[IBIS Ver]   4.2
[File Name]  stm32f2_wlcsp64.ibs
[File Rev]   1.0
[Date]   31-Aug-2011
[Source]   STMicroelectronics NV
[Notes]   The I/O models have been made by simulation and qualified
   with recomandation of QualityIBIS flow.
   Some Models, library and pin names may be modified.
   Details of modified names can be found below.
ORIGINAL NAME   ::  MODIFIED NAME   :: COMMENTS(if any)
IO8USB_LSFS_OTG_FT  ::  IO8USB_LSFS_OTG_FT_USB   :: Model in USB mode.
IO8USB_LSFS_OTG_FT  ::  IO8USB_LSFS_OTG_FT_NON_USB_DNV33  :: Model in other than USB mode & pad pin = DNV33
IO8USB_LSFS_OTG_FT  ::  IO8USB_LSFS_OTG_FT_NON_USB_DPV33  :: Model in other than USB mode & pad pin = DPV33
[Disclaimer] These IBIS models are the proprietary information of
   STMicroelectronics and are disclosed to users solely for
   modeling and simulation purposes. No further license is
   implied. All warranties express, implied, or statutory,
   including any implied warranty of fitness for a particular
   purpose or implied warranty against infringement, are
   hereby disclaimed. STMicroelectronics reserves the right
   to change the IBIS models at any time and without notice.
[Copyright]  (c) STMicroelectronics
   All rights reserved. Reproduction in whole or part is prohibited
   without the written consent of the copyright holder.
[Component]  STM32F2_WLCSP
[Manufacturer] STMicroelectronics NV
[Package]
| variable   typ   min   max
R_pkg   0.000mOhm   0.000mOhm   0.000mOhm
L_pkg   0.000nH   0.000nH   0.000nH
C_pkg   0.000pF   0.000pF   0.000pF
[Pin]   signal_name   model_name
|- PE2 IO8PROG2M25M50M100M_ARSUDQ_FT
|- PE3 IO8PROG2M25M50M100M_ARSUDQ_FT
|- PE4 IO8PROG2M25M50M100M_ARSUDQ_FT
|- PE5 IO8PROG2M25M50M100M_ARSUDQ_FT
|- PE6 IO8PROG2M25M50M100M_ARSUDQ_FT
|A9 VBAT VDD33IOSWCO_MOSSWI_FT
B8 PC13 IO8PROG2M25M50M100M_ARWSUDQ_FT_V33
B9 PC14 IO8PROG2M25M50M100M_ARWSUDQ_FT
C9 PC15 IO8PROG2M25M50M100M_ARSUDQ_FT
|- VSS_5 VSSIOCO
|- VDD_5 VDD33IOCO
E9 PH0 IO8PROG2M25M50M100M_ARSUDQ_FT
F9 PH1 IO8PROG2M25M50M100M_ARSUDQ_FT
|E8 NRST RESET
G9 PC0 IO8PROG2M25M50M100M_AR3WSUDQ_FT
F8 PC1 IO8PROG2M25M50M100M_AR3WSUDQ_FT
D7 PC2 IO8PROG2M25M50M100M_AR3WSUDQ_FT
G8 PC3 IO8PROG2M25M50M100M_AR3WSUDQ_FT
|- VDD_12 VDD33IOCO_VSSIOCO_MOSSWI_FT
|- VSSA VSSCO
|F7 VREF+ VDD33CO
|- VDDA VDD33CO
E7 PA0 IO8PROG2M25M50M100M_AR3WSUDQ_FT_V33
H8 PA1 IO8PROG2M25M50M100M_AR3WSUDQ_FT
J9 PA2 IO8PROG2M25M50M100M_AR3WSUDQ_FT
G7 PA3 IO8PROG2M25M50M100M_AR3WSUDQ_FT
|F1 VSS_4 VSSIOCO
|H7 REGOFF VSSIOCO
|E1 VDD_4 VDD33IOCO
J8 PA4 IO8PROG2M25M50M100M_AR3WSUDQ_FT
H6 PA5 IO8PROG2M25M50M100M_AR3WSUDQ_FT
H5 PA6 IO8PROG2M25M50M100M_AR3WSUDQ_FT
J7 PA7 IO8PROG2M25M50M100M_AR3WSUDQ_FT
H4 PC4 IO8PROG2M25M50M100M_AR3WSUDQ_FT
G3 PC5 IO8PROG2M25M50M100M_AR3WSUDQ_FT
J6 PB0 IO8PROG2M25M50M100M_AR3WSUDQ_FT
J5 PB1 IO8PROG2M25M50M100M_AR3WSUDQ_FT
J4 PB2 IO8PROG2M25M50M100M_AR3WSUDQ_FT
|- PE7 IO8PROG2M25M50M100M_ARSUDQ_FT
|- PE8 IO8PROG2M25M50M100M_ARSUDQ_FT
|- PE9 IO8PROG2M25M50M100M_ARSUDQ_FT
|- PE10 IO8PROG2M25M50M100M_ARSUDQ_FT
|- PE11 IO8PROG2M25M50M100M_ARSUDQ_FT
|- PE12 IO8PROG2M25M50M100M_ARSUDQ_FT
|- PE13 IO8PROG2M25M50M100M_ARSUDQ_FT
|- PE14 IO8PROG2M25M50M100M_ARSUDQ_FT
|- PE15 IO8PROG2M25M50M100M_ARSUDQ_FT
H3 PB10 IO8PROG2M25M50M100M_ARSUDQ_I2CIN_FT
J2 PB11 IO8PROG2M25M50M100M_ARSUDQ_I2CIN_FT
|J3 VCAP1_0
|- VDD_1
J1 PB12 IO8USB_ID_OTG_FT
H2 PB13 IO8USB_VBUS_OTG_FT
|H1 PA11 IO8USB_LSFS_OTG_FT_USB
H1 PA11 IO8USB_LSFS_OTG_FT_NON_USB_DNV33
|G1 PA12 IO8USB_LSFS_OTG_FT_USB
G1 PA12 IO8USB_LSFS_OTG_FT_NON_USB_DPV33
|- PD8 IO8PROG2M25M50M100M_ARSUDQ_FT
|- PD9 IO8PROG2M25M50M100M_ARSUDQ_FT
|- PD10 IO8PROG2M25M50M100M_ARSUDQ_FT
|- PD11 IO8PROG2M25M50M100M_ARSUDQ_FT
|- PD12 IO8PROG2M25M50M100M_ARSUDQ_FT
|- PD13 IO8PROG2M25M50M100M_ARSUDQ_FT
|- PD14 IO8PROG2M25M50M100M_ARSUDQ_FT
|- PD15 IO8PROG2M25M50M100M_ARSUDQ_FT
G2 PC6 IO8PROG2M25M50M100M_ARSUDQ_FT
F2 PC7 IO8PROG2M25M50M100M_ARSUDQ_FT
F3 PC8 IO8PROG2M25M50M100M_ARSUDQ_FT
D1 PC9 IO8PROG2M25M50M100M_ARSUDQ_I2CIN_FT
E2 PA8 IO8PROG2M25M50M100M_ARSUDQ_I2CIN_FT
E3 PA9 IO8USB_VBUS_OTG_FT
D3 PA10 IO8USB_ID_OTG_FT
D2 PA11 IO8USB_LSFS_OTG_FT_USB
|D2 PA11 IO8USB_LSFS_OTG_FT_NON_USB_DNV33
C1 PA12 IO8USB_LSFS_OTG_FT_USB
|C1 PA12 IO8USB_LSFS_OTG_FT_NON_USB_DPV33
B2 PA13 IO8PROG2M25M50M100M_ARSUDQ_FT
|C2 VCAP2
|B1 VSS_2
|A8 VDD_2
A1 PA14 IO8PROG2M25M50M100M_ARSUDQ_FT
A2 PA15 IO8PROG2M25M50M100M_AR3WSUDQ_FT
B3 PC10 IO8PROG2M25M50M100M_ARSUDQ_FT
C3 PC11 IO8PROG2M25M50M100M_ARSUDQ_FT
A3 PC12 IO8PROG2M25M50M100M_ARSUDQ_FT
|- PD0 IO8PROG2M25M50M100M_ARSUDQ_FT
|- PD1 IO8PROG2M25M50M100M_ARSUDQ_FT
C7 PD2 IO8PROG2M25M50M100M_ARSUDQ_FT
|- PD3 IO8PROG2M25M50M100M_ARSUDQ_FT
|- PD4 IO8PROG2M25M50M100M_ARSUDQ_FT
|- PD5 IO8PROG2M25M50M100M_ARSUDQ_FT
|- PD6 IO8PROG2M25M50M100M_ARSUDQ_FT
|- PD7 IO8PROG2M25M50M100M_ARSUDQ_FT
A4 PB3 IO8PROG2M25M50M100M_ARSUDQ_FT
B4 PB4 IO8PROG2M25M50M100M_ARSUDQ_FT
A5 PB5 IO8PROG2M25M50M100M_AR3WSUDQ_FT
B5 PB6 IO8PROG2M25M50M100M_ARSUDQ_I2CIN_FT
A6 PB7 IO8PROG2M25M50M100M_ARSUDQ_I2CIN_FT
B6 BOOT0 VPP_TEST_HV
B7 PB8 IO8PROG2M25M50M100M_ARSUDQ_I2CIN_FT
A7 PB9 IO8PROG2M25M50M100M_ARSUDQ_I2CIN_FT
|- PE0 IO8PROG2M25M50M100M_ARSUDQ_FT
|- PE1 IO8PROG2M25M50M100M_ARSUDQ_FT
|- NC
|D8 VSS_3
|D9 VDD_3  VDD33CO
[Diff Pin]  inv_pin   vdiff tdelay_typ tdelay_min tdelay_max
H1 G1 200mV 0  0 0
D2 C1 200mV 0  0 0
[Model Selector] IO8PROG2M25M50M100M_AR3WSUDQ_FT_V33
IO8PROG2M25M50M100M_AR3WSUDQ_DRV_V33_00   DRIVER MODEL  : SPEEDAV33=0 SPEEDBV33=0
IO8PROG2M25M50M100M_AR3WSUDQ_DRV_V33_01   DRIVER MODEL  : SPEEDAV33=0 SPEEDBV33=1
IO8PROG2M25M50M100M_AR3WSUDQ_DRV_V33_10   DRIVER MODEL  : SPEEDAV33=1 SPEEDBV33=0
IO8PROG2M25M50M100M_AR3WSUDQ_DRV_V33_11   DRIVER MODEL  : SPEEDAV33=1 SPEEDBV33=1
IO8PROG2M25M50M100M_AR3WSUDQ_RCV_V33_0   CMOS RECIEVER : ENHYSV33=0  OUTPUT=ZIV33
IO8PROG2M25M50M100M_AR3WSUDQ_RCV_V33_0_T  TTL  RECIEVER : ENHYSV33=0  OUTPUT=ZIV33
IO8PROG2M25M50M100M_AR3WSUDQ_RCV_V33_1   CMOS RECIEVER : ENHYSV33=1  OUTPUT=ZIV33
IO8PROG2M25M50M100M_AR3WSUDQ_RCV_V33_1_T  TTL  RECIEVER : ENHYSV33=1  OUTPUT=ZIV33
[Model Selector] IO8PROG2M25M50M100M_AR3WSUDQ_FT
IO8PROG2M25M50M100M_AR3WSUDQ_FT_DRV_00   DRIVER MODEL  : SPEEDAV12=0 SPEEDBV12=0
IO8PROG2M25M50M100M_AR3WSUDQ_FT_DRV_01   DRIVER MODEL  : SPEEDAV12=0 SPEEDBV12=1
IO8PROG2M25M50M100M_AR3WSUDQ_FT_DRV_10   DRIVER MODEL  : SPEEDAV12=1 SPEEDBV12=0
IO8PROG2M25M50M100M_AR3WSUDQ_FT_DRV_11   DRIVER MODEL  : SPEEDAV12=1 SPEEDBV12=1
IO8PROG2M25M50M100M_AR3WSUDQ_FT_RCV_00   CMOS RECIEVER : ENHYSV12=0  OUTPUT=ZIV12
IO8PROG2M25M50M100M_AR3WSUDQ_FT_RCV_00_T  TTL  RECIEVER : ENHYSV12=0  OUTPUT=ZIV12
IO8PROG2M25M50M100M_AR3WSUDQ_FT_RCV_01   CMOS RECIEVER : ENHYSV12=0  OUTPUT=ZIV33
IO8PROG2M25M50M100M_AR3WSUDQ_FT_RCV_01_T  TTL  RECIEVER : ENHYSV12=0  OUTPUT=ZIV33
IO8PROG2M25M50M100M_AR3WSUDQ_FT_RCV_10   CMOS RECIEVER : ENHYSV12=1  OUTPUT=ZIV12
IO8PROG2M25M50M100M_AR3WSUDQ_FT_RCV_10_T  TTL  RECIEVER : ENHYSV12=1  OUTPUT=ZIV12
IO8PROG2M25M50M100M_AR3WSUDQ_FT_RCV_11   CMOS RECIEVER : ENHYSV12=1  OUTPUT=ZIV33
IO8PROG2M25M50M100M_AR3WSUDQ_FT_RCV_11_T  TTL  RECIEVER : ENHYSV12=1  OUTPUT=ZIV33
[Model Selector] IO8PROG2M25M50M100M_ARSUDQ_FT
IO8PROG2M25M50M100M_ARSUDQ_FT_DRV_00   DRIVER MODEL  : SPEEDAV12=0 SPEEDBV12=0
IO8PROG2M25M50M100M_ARSUDQ_FT_DRV_01   DRIVER MODEL  : SPEEDAV12=0 SPEEDBV12=1
IO8PROG2M25M50M100M_ARSUDQ_FT_DRV_10   DRIVER MODEL  : SPEEDAV12=1 SPEEDBV12=0
IO8PROG2M25M50M100M_ARSUDQ_FT_DRV_11   DRIVER MODEL  : SPEEDAV12=1 SPEEDBV12=1
IO8PROG2M25M50M100M_ARSUDQ_FT_RCV_00   CMOS RECIEVER : ENHYSV12=0  OUTPUT=ZIV12
IO8PROG2M25M50M100M_ARSUDQ_FT_RCV_00_T   TTL  RECIEVER : ENHYSV12=0  OUTPUT=ZIV12
IO8PROG2M25M50M100M_ARSUDQ_FT_RCV_01   CMOS RECIEVER : ENHYSV12=0  OUTPUT=ZIV33
IO8PROG2M25M50M100M_ARSUDQ_FT_RCV_01_T   TTL  RECIEVER : ENHYSV12=0  OUTPUT=ZIV33
IO8PROG2M25M50M100M_ARSUDQ_FT_RCV_10   CMOS RECIEVER : ENHYSV12=1  OUTPUT=ZIV12
IO8PROG2M25M50M100M_ARSUDQ_FT_RCV_10_T   TTL  RECIEVER : ENHYSV12=1  OUTPUT=ZIV12
IO8PROG2M25M50M100M_ARSUDQ_FT_RCV_11   CMOS RECIEVER : ENHYSV12=1  OUTPUT=ZIV33
IO8PROG2M25M50M100M_ARSUDQ_FT_RCV_11_T   TTL  RECIEVER : ENHYSV12=1  OUTPUT=ZIV33
[Model Selector] IO8PROG2M25M50M100M_ARSUDQ_I2CIN_FT
IO8PROG2M25M50M100M_ARSUDQ_I2CIN_DRV_00   DRIVER MODEL  : SPEEDAV12=0 SPEEDBV12=0
IO8PROG2M25M50M100M_ARSUDQ_I2CIN_DRV_01   DRIVER MODEL  : SPEEDAV12=0 SPEEDBV12=1
IO8PROG2M25M50M100M_ARSUDQ_I2CIN_DRV_10   DRIVER MODEL  : SPEEDAV12=1 SPEEDBV12=0
IO8PROG2M25M50M100M_ARSUDQ_I2CIN_DRV_11   DRIVER MODEL  : SPEEDAV12=1 SPEEDBV12=1
IO8PROG2M25M50M100M_I2CIN_RCV_ZII2C_00   CMOS RECIEVER : TESTI2CV12=0  HSFSV12=0
IO8PROG2M25M50M100M_I2CIN_RCV_ZII2C_00_T   TTL  RECIEVER : TESTI2CV12=0  HSFSV12=0
IO8PROG2M25M50M100M_I2CIN_RCV_ZII2C_01   CMOS RECIEVER : TESTI2CV12=0  HSFSV12=1
IO8PROG2M25M50M100M_I2CIN_RCV_ZII2C_01_T   TTL  RECIEVER : TESTI2CV12=0  HSFSV12=1
IO8PROG2M25M50M100M_I2CIN_RCV_ZII2C_10   CMOS RECIEVER : TESTI2CV12=1  HSFSV12=0
IO8PROG2M25M50M100M_I2CIN_RCV_ZII2C_10_T   TTL  RECIEVER : TESTI2CV12=1  HSFSV12=0
IO8PROG2M25M50M100M_I2CIN_RCV_ZII2C_11   CMOS RECIEVER : TESTI2CV12=1  HSFSV12=1
IO8PROG2M25M50M100M_I2CIN_RCV_ZII2C_11_T   TTL  RECIEVER : TESTI2CV12=1  HSFSV12=1
IO8PROG2M25M50M100M_I2CIN_RCV_ZIV12_0   CMOS RECIEVER : ENHYSV12=0  OUTPUT=ZIV12
IO8PROG2M25M50M100M_I2CIN_RCV_ZIV12_0_T   TTL  RECIEVER : ENHYSV12=0  OUTPUT=ZIV12
IO8PROG2M25M50M100M_I2CIN_RCV_ZIV12_1   CMOS RECIEVER : ENHYSV12=1  OUTPUT=ZIV12
IO8PROG2M25M50M100M_I2CIN_RCV_ZIV12_1_T   TTL  RECIEVER : ENHYSV12=1  OUTPUT=ZIV12
IO8PROG2M25M50M100M_I2CIN_RCV_ZIV33_0   CMOS RECIEVER : ENHYSV12=0  OUTPUT=ZIV33
IO8PROG2M25M50M100M_I2CIN_RCV_ZIV33_0_T   TTL  RECIEVER : ENHYSV12=0  OUTPUT=ZIV33
IO8PROG2M25M50M100M_I2CIN_RCV_ZIV33_1   CMOS RECIEVER : ENHYSV12=1  OUTPUT=ZIV33
IO8PROG2M25M50M100M_I2CIN_RCV_ZIV33_1_T   TTL  RECIEVER : ENHYSV12=1  OUTPUT=ZIV33
[Model Selector] IO8PROG2M25M50M100M_ARWSUDQ_FT_V33
IO8PROG2M25M50M100M_ARWSUDQ_DRV_V33_00   DRIVER MODEL  : SPEEDAV33=0 SPEEDBV33=0
IO8PROG2M25M50M100M_ARWSUDQ_DRV_V33_01   DRIVER MODEL  : SPEEDAV33=0 SPEEDBV33=1
IO8PROG2M25M50M100M_ARWSUDQ_DRV_V33_10   DRIVER MODEL  : SPEEDAV33=1 SPEEDBV33=0
IO8PROG2M25M50M100M_ARWSUDQ_DRV_V33_11   DRIVER MODEL  : SPEEDAV33=1 SPEEDBV33=1
IO8PROG2M25M50M100M_ARWSUDQ_RCV_V33_0   CMOS RECIEVER : ENHYSV33=0  OUTPUT=ZIV33
IO8PROG2M25M50M100M_ARWSUDQ_RCV_V33_0_T   TTL  RECIEVER : ENHYSV33=0  OUTPUT=ZIV33
IO8PROG2M25M50M100M_ARWSUDQ_RCV_V33_1   CMOS RECIEVER : ENHYSV33=1  OUTPUT=ZIV33
IO8PROG2M25M50M100M_ARWSUDQ_RCV_V33_1_T   TTL  RECIEVER : ENHYSV33=1  OUTPUT=ZIV33
[Model Selector] IO8PROG2M25M50M100M_ARWSUDQ_FT
IO8PROG2M25M50M100M_ARWSUDQ_FT_DRV_00   DRIVER MODEL  : SPEEDAV12=0 SPEEDBV12=0
IO8PROG2M25M50M100M_ARWSUDQ_FT_DRV_01   DRIVER MODEL  : SPEEDAV12=0 SPEEDBV12=1
IO8PROG2M25M50M100M_ARWSUDQ_FT_DRV_10   DRIVER MODEL  : SPEEDAV12=1 SPEEDBV12=0
IO8PROG2M25M50M100M_ARWSUDQ_FT_DRV_11   DRIVER MODEL  : SPEEDAV12=1 SPEEDBV12=1
IO8PROG2M25M50M100M_ARWSUDQ_FT_RCV_00   CMOS RECIEVER : ENHYSV12=0  OUTPUT=ZIV12
IO8PROG2M25M50M100M_ARWSUDQ_FT_RCV_00_T   TTL  RECIEVER : ENHYSV12=0  OUTPUT=ZIV12
IO8PROG2M25M50M100M_ARWSUDQ_FT_RCV_01   CMOS RECIEVER : ENHYSV12=0  OUTPUT=ZIV33
IO8PROG2M25M50M100M_ARWSUDQ_FT_RCV_01_T   TTL  RECIEVER : ENHYSV12=0  OUTPUT=ZIV33
IO8PROG2M25M50M100M_ARWSUDQ_FT_RCV_10   CMOS RECIEVER : ENHYSV12=1  OUTPUT=ZIV12
IO8PROG2M25M50M100M_ARWSUDQ_FT_RCV_10_T   TTL  RECIEVER : ENHYSV12=1  OUTPUT=ZIV12
IO8PROG2M25M50M100M_ARWSUDQ_FT_RCV_11   CMOS RECIEVER : ENHYSV12=1  OUTPUT=ZIV33
IO8PROG2M25M50M100M_ARWSUDQ_FT_RCV_11_T   TTL  RECIEVER : ENHYSV12=1  OUTPUT=ZIV33
[Model Selector] IO8USB_ID_OTG_FT
IO8USB_ID_OTG_FT_DRV_00   DRIVER MODEL  : SPEEDAV12=0 SPEEDBV12=0
IO8USB_ID_OTG_FT_DRV_01   DRIVER MODEL  : SPEEDAV12=0 SPEEDBV12=1
IO8USB_ID_OTG_FT_DRV_10   DRIVER MODEL  : SPEEDAV12=1 SPEEDBV12=0
IO8USB_ID_OTG_FT_DRV_11   DRIVER MODEL  : SPEEDAV12=1 SPEEDBV12=1
IO8USB_ID_OTG_FT_RCV_00   CMOS RECIEVER : ENHYSV12=0  OUTPUT=ZIV12
IO8USB_ID_OTG_FT_RCV_00_T   TTL  RECIEVER : ENHYSV12=0  OUTPUT=ZIV12
IO8USB_ID_OTG_FT_RCV_01   CMOS RECIEVER : ENHYSV12=0  OUTPUT=ZIV33
IO8USB_ID_OTG_FT_RCV_01_T   TTL  RECIEVER : ENHYSV12=0  OUTPUT=ZIV33
IO8USB_ID_OTG_FT_RCV_10   CMOS RECIEVER : ENHYSV12=1  OUTPUT=ZIV12
IO8USB_ID_OTG_FT_RCV_10_T   TTL  RECIEVER : ENHYSV12=1  OUTPUT=ZIV12
IO8USB_ID_OTG_FT_RCV_11   CMOS RECIEVER : ENHYSV12=1  OUTPUT=ZIV33
IO8USB_ID_OTG_FT_RCV_11_T   TTL  RECIEVER : ENHYSV12=1  OUTPUT=ZIV33
[Model Selector] IO8USB_LSFS_OTG_FT_USB
IO8USB_LSFS_OTG_FT_DRV_USB_0   DRIVER : USBLSFSV12=0 ENUSBV12=0
IO8USB_LSFS_OTG_FT_DRV_USB_1   DRIVER : USBLSFSV12=1 ENUSBV12=0
IO8USB_LSFS_OTG_FT_RCV_USB   USB  RECIEVER : ENHYSV12=1  OUTPUT=USBZIV12
[Model Selector] IO8USB_LSFS_OTG_FT_NON_USB_DNV33
IO8USB_LSFS_OTG_FT_DRV_IO8_DNV33_00   DRIVER : SPEEDAV12=0 SPEEDBV12=0 ENUSBV12=1
IO8USB_LSFS_OTG_FT_DRV_IO8_DNV33_01   DRIVER : SPEEDAV12=0 SPEEDBV12=1 ENUSBV12=1
IO8USB_LSFS_OTG_FT_DRV_IO8_DNV33_10   DRIVER : SPEEDAV12=1 SPEEDBV12=0 ENUSBV12=1
IO8USB_LSFS_OTG_FT_DRV_IO8_DNV33_11   DRIVER : SPEEDAV12=1 SPEEDBV12=1 ENUSBV12=1
IO8USB_LSFS_OTG_FT_RCV_IO8_ZINV12_0   CMOS RECIEVER : ENHYSV12=0  OUTPUT=ZIV12
IO8USB_LSFS_OTG_FT_RCV_IO8_ZINV12_0_T  TTL  RECIEVER : ENHYSV12=0  OUTPUT=ZIV12
IO8USB_LSFS_OTG_FT_RCV_IO8_ZINV12_1   CMOS RECIEVER : ENHYSV12=1  OUTPUT=ZIV12
IO8USB_LSFS_OTG_FT_RCV_IO8_ZINV12_1_T  TTL  RECIEVER : ENHYSV12=1  OUTPUT=ZIV12
IO8USB_LSFS_OTG_FT_RCV_IO8_ZINV33_0   CMOS RECIEVER : ENHYSV12=0  OUTPUT=ZIV33
IO8USB_LSFS_OTG_FT_RCV_IO8_ZINV33_0_T  TTL  RECIEVER : ENHYSV12=0  OUTPUT=ZIV33
IO8USB_LSFS_OTG_FT_RCV_IO8_ZINV33_1   CMOS RECIEVER : ENHYSV12=1  OUTPUT=ZIV33
IO8USB_LSFS_OTG_FT_RCV_IO8_ZINV33_1_T  TTL  RECIEVER : ENHYSV12=1  OUTPUT=ZIV33
[Model Selector] IO8USB_LSFS_OTG_FT_NON_USB_DPV33
IO8USB_LSFS_OTG_FT_DRV_IO8_DPV33_00   DRIVER : SPEEDAV12=0 SPEEDBV12=0 ENUSBV12=1
IO8USB_LSFS_OTG_FT_DRV_IO8_DPV33_01   DRIVER : SPEEDAV12=0 SPEEDBV12=1 ENUSBV12=1
IO8USB_LSFS_OTG_FT_DRV_IO8_DPV33_10   DRIVER : SPEEDAV12=1 SPEEDBV12=0 ENUSBV12=1
IO8USB_LSFS_OTG_FT_DRV_IO8_DPV33_11   DRIVER : SPEEDAV12=1 SPEEDBV12=1 ENUSBV12=1
IO8USB_LSFS_OTG_FT_RCV_IO8_ZIPV12_0   CMOS RECIEVER : ENHYSV12=0  OUTPUT=ZIV12
IO8USB_LSFS_OTG_FT_RCV_IO8_ZIPV12_0_T  TTL  RECIEVER : ENHYSV12=0  OUTPUT=ZIV12
IO8USB_LSFS_OTG_FT_RCV_IO8_ZIPV12_1   CMOS RECIEVER : ENHYSV12=1  OUTPUT=ZIV12
IO8USB_LSFS_OTG_FT_RCV_IO8_ZIPV12_1_T  TTL  RECIEVER : ENHYSV12=1  OUTPUT=ZIV12
IO8USB_LSFS_OTG_FT_RCV_IO8_ZIPV33_0   CMOS RECIEVER : ENHYSV12=0  OUTPUT=ZIV33
IO8USB_LSFS_OTG_FT_RCV_IO8_ZIPV33_0_T  TTL  RECIEVER : ENHYSV12=0  OUTPUT=ZIV33
IO8USB_LSFS_OTG_FT_RCV_IO8_ZIPV33_1   CMOS RECIEVER : ENHYSV12=1  OUTPUT=ZIV33
IO8USB_LSFS_OTG_FT_RCV_IO8_ZIPV33_1_T  TTL  RECIEVER : ENHYSV12=1  OUTPUT=ZIV33
[Model Selector] IO8USB_VBUS_OTG_FT
IO8USB_VBUS_OTG_FT_DRV_00   DRIVER MODEL  : SPEEDAV12=0 SPEEDBV12=0
IO8USB_VBUS_OTG_FT_DRV_01   DRIVER MODEL  : SPEEDAV12=0 SPEEDBV12=1
IO8USB_VBUS_OTG_FT_DRV_10   DRIVER MODEL  : SPEEDAV12=1 SPEEDBV12=0
IO8USB_VBUS_OTG_FT_DRV_11   DRIVER MODEL  : SPEEDAV12=1 SPEEDBV12=1
IO8USB_VBUS_OTG_FT_RCV_00   CMOS RECIEVER : ENHYSV12=0  OUTPUT=ZIV12
IO8USB_VBUS_OTG_FT_RCV_00_T   TTL  RECIEVER : ENHYSV12=0  OUTPUT=ZIV12
IO8USB_VBUS_OTG_FT_RCV_01   CMOS RECIEVER : ENHYSV12=0  OUTPUT=ZIV33
IO8USB_VBUS_OTG_FT_RCV_01_T   TTL  RECIEVER : ENHYSV12=0  OUTPUT=ZIV33
IO8USB_VBUS_OTG_FT_RCV_10   CMOS RECIEVER : ENHYSV12=1  OUTPUT=ZIV12
IO8USB_VBUS_OTG_FT_RCV_10_T   TTL  RECIEVER : ENHYSV12=1  OUTPUT=ZIV12
IO8USB_VBUS_OTG_FT_RCV_11   CMOS RECIEVER : ENHYSV12=1  OUTPUT=ZIV33
IO8USB_VBUS_OTG_FT_RCV_11_T   TTL  RECIEVER : ENHYSV12=1  OUTPUT=ZIV33
[Model Selector] VPP_TEST_HV
VPP_TEST_HV_00   CMOS RECIEVER : ENHYSV12=0  OUTPUT=ZIV12
VPP_TEST_HV_00_T   TTL  RECIEVER : ENHYSV12=0  OUTPUT=ZIV12
VPP_TEST_HV_01   CMOS RECIEVER : ENHYSV12=0  OUTPUT=ZIV33
VPP_TEST_HV_01_T   TTL  RECIEVER : ENHYSV12=0  OUTPUT=ZIV33
VPP_TEST_HV_10   CMOS RECIEVER : ENHYSV12=1  OUTPUT=ZIV12
VPP_TEST_HV_10_T   TTL  RECIEVER : ENHYSV12=1  OUTPUT=ZIV12
VPP_TEST_HV_11   CMOS RECIEVER : ENHYSV12=1  OUTPUT=ZIV33
VPP_TEST_HV_11_T   TTL  RECIEVER : ENHYSV12=1  OUTPUT=ZIV33
| Models and submodels in the file (131): IO8PROG2M25M50M100M_AR3WSUDQ_DRV_V33_00 (3-state), IO8PROG2M25M50M100M_AR3WSUDQ_DRV_V33_01 (3-state), IO8PROG2M25M50M100M_AR3WSUDQ_DRV_V33_10 (3-state), IO8PROG2M25M50M100M_AR3WSUDQ_DRV_V33_11 (3-state), IO8PROG2M25M50M100M_AR3WSUDQ_FT_DRV_00 (3-state), IO8PROG2M25M50M100M_AR3WSUDQ_FT_DRV_01 (3-state), IO8PROG2M25M50M100M_AR3WSUDQ_FT_DRV_10 (3-state), IO8PROG2M25M50M100M_AR3WSUDQ_FT_DRV_11 (3-state), IO8PROG2M25M50M100M_AR3WSUDQ_FT_RCV_00 (Input), IO8PROG2M25M50M100M_AR3WSUDQ_FT_RCV_00_T (Input), IO8PROG2M25M50M100M_AR3WSUDQ_FT_RCV_01 (Input), IO8PROG2M25M50M100M_AR3WSUDQ_FT_RCV_01_T (Input), IO8PROG2M25M50M100M_AR3WSUDQ_FT_RCV_10 (Input), IO8PROG2M25M50M100M_AR3WSUDQ_FT_RCV_10_T (Input), IO8PROG2M25M50M100M_AR3WSUDQ_FT_RCV_11 (Input), IO8PROG2M25M50M100M_AR3WSUDQ_FT_RCV_11_T (Input), IO8PROG2M25M50M100M_AR3WSUDQ_RCV_V33_0 (Input), IO8PROG2M25M50M100M_AR3WSUDQ_RCV_V33_0_T (Input), IO8PROG2M25M50M100M_AR3WSUDQ_RCV_V33_1 (Input), IO8PROG2M25M50M100M_AR3WSUDQ_RCV_V33_1_T (Input), IO8PROG2M25M50M100M_ARSUDQ_FT_DRV_00 (3-state), IO8PROG2M25M50M100M_ARSUDQ_FT_DRV_01 (3-state), IO8PROG2M25M50M100M_ARSUDQ_FT_DRV_10 (3-state), IO8PROG2M25M50M100M_ARSUDQ_FT_DRV_11 (3-state), IO8PROG2M25M50M100M_ARSUDQ_FT_RCV_00 (Input), IO8PROG2M25M50M100M_ARSUDQ_FT_RCV_00_T (Input), IO8PROG2M25M50M100M_ARSUDQ_FT_RCV_01 (Input), IO8PROG2M25M50M100M_ARSUDQ_FT_RCV_01_T (Input), IO8PROG2M25M50M100M_ARSUDQ_FT_RCV_10 (Input), IO8PROG2M25M50M100M_ARSUDQ_FT_RCV_10_T (Input), IO8PROG2M25M50M100M_ARSUDQ_FT_RCV_11 (Input), IO8PROG2M25M50M100M_ARSUDQ_FT_RCV_11_T (Input), IO8PROG2M25M50M100M_ARSUDQ_I2CIN_DRV_00 (3-state), IO8PROG2M25M50M100M_ARSUDQ_I2CIN_DRV_01 (3-state), IO8PROG2M25M50M100M_ARSUDQ_I2CIN_DRV_10 (3-state), IO8PROG2M25M50M100M_ARSUDQ_I2CIN_DRV_11 (3-state), IO8PROG2M25M50M100M_ARWSUDQ_DRV_V33_00 (3-state), IO8PROG2M25M50M100M_ARWSUDQ_DRV_V33_01 (3-state), IO8PROG2M25M50M100M_ARWSUDQ_DRV_V33_10 (3-state), IO8PROG2M25M50M100M_ARWSUDQ_DRV_V33_11 (3-state), IO8PROG2M25M50M100M_ARWSUDQ_FT_DRV_00 (3-state), IO8PROG2M25M50M100M_ARWSUDQ_FT_DRV_01 (3-state), IO8PROG2M25M50M100M_ARWSUDQ_FT_DRV_10 (3-state), IO8PROG2M25M50M100M_ARWSUDQ_FT_DRV_11 (3-state), IO8PROG2M25M50M100M_ARWSUDQ_FT_RCV_00 (Input), IO8PROG2M25M50M100M_ARWSUDQ_FT_RCV_00_T (Input), IO8PROG2M25M50M100M_ARWSUDQ_FT_RCV_01 (Input), IO8PROG2M25M50M100M_ARWSUDQ_FT_RCV_01_T (Input), IO8PROG2M25M50M100M_ARWSUDQ_FT_RCV_10 (Input), IO8PROG2M25M50M100M_ARWSUDQ_FT_RCV_10_T (Input), IO8PROG2M25M50M100M_ARWSUDQ_FT_RCV_11 (Input), IO8PROG2M25M50M100M_ARWSUDQ_FT_RCV_11_T (Input), IO8PROG2M25M50M100M_ARWSUDQ_RCV_V33_0 (Input), IO8PROG2M25M50M100M_ARWSUDQ_RCV_V33_0_T (Input), IO8PROG2M25M50M100M_ARWSUDQ_RCV_V33_1 (Input), IO8PROG2M25M50M100M_ARWSUDQ_RCV_V33_1_T (Input), IO8PROG2M25M50M100M_I2CIN_RCV_ZII2C_00 (Input), IO8PROG2M25M50M100M_I2CIN_RCV_ZII2C_00_T (Input), IO8PROG2M25M50M100M_I2CIN_RCV_ZII2C_01 (Input), IO8PROG2M25M50M100M_I2CIN_RCV_ZII2C_01_T (Input), IO8PROG2M25M50M100M_I2CIN_RCV_ZII2C_10 (Input), IO8PROG2M25M50M100M_I2CIN_RCV_ZII2C_10_T (Input), IO8PROG2M25M50M100M_I2CIN_RCV_ZII2C_11 (Input), IO8PROG2M25M50M100M_I2CIN_RCV_ZII2C_11_T (Input), IO8PROG2M25M50M100M_I2CIN_RCV_ZIV12_0 (Input), IO8PROG2M25M50M100M_I2CIN_RCV_ZIV12_0_T (Input), IO8PROG2M25M50M100M_I2CIN_RCV_ZIV12_1 (Input), IO8PROG2M25M50M100M_I2CIN_RCV_ZIV12_1_T (Input), IO8PROG2M25M50M100M_I2CIN_RCV_ZIV33_0 (Input), IO8PROG2M25M50M100M_I2CIN_RCV_ZIV33_0_T (Input), IO8PROG2M25M50M100M_I2CIN_RCV_ZIV33_1 (Input), IO8PROG2M25M50M100M_I2CIN_RCV_ZIV33_1_T (Input), IO8USB_ID_OTG_FT_DRV_00 (3-state), IO8USB_ID_OTG_FT_DRV_01 (3-state), IO8USB_ID_OTG_FT_DRV_10 (3-state), IO8USB_ID_OTG_FT_DRV_11 (3-state), IO8USB_ID_OTG_FT_RCV_00 (Input), IO8USB_ID_OTG_FT_RCV_00_T (Input), IO8USB_ID_OTG_FT_RCV_01 (Input), IO8USB_ID_OTG_FT_RCV_01_T (Input)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
